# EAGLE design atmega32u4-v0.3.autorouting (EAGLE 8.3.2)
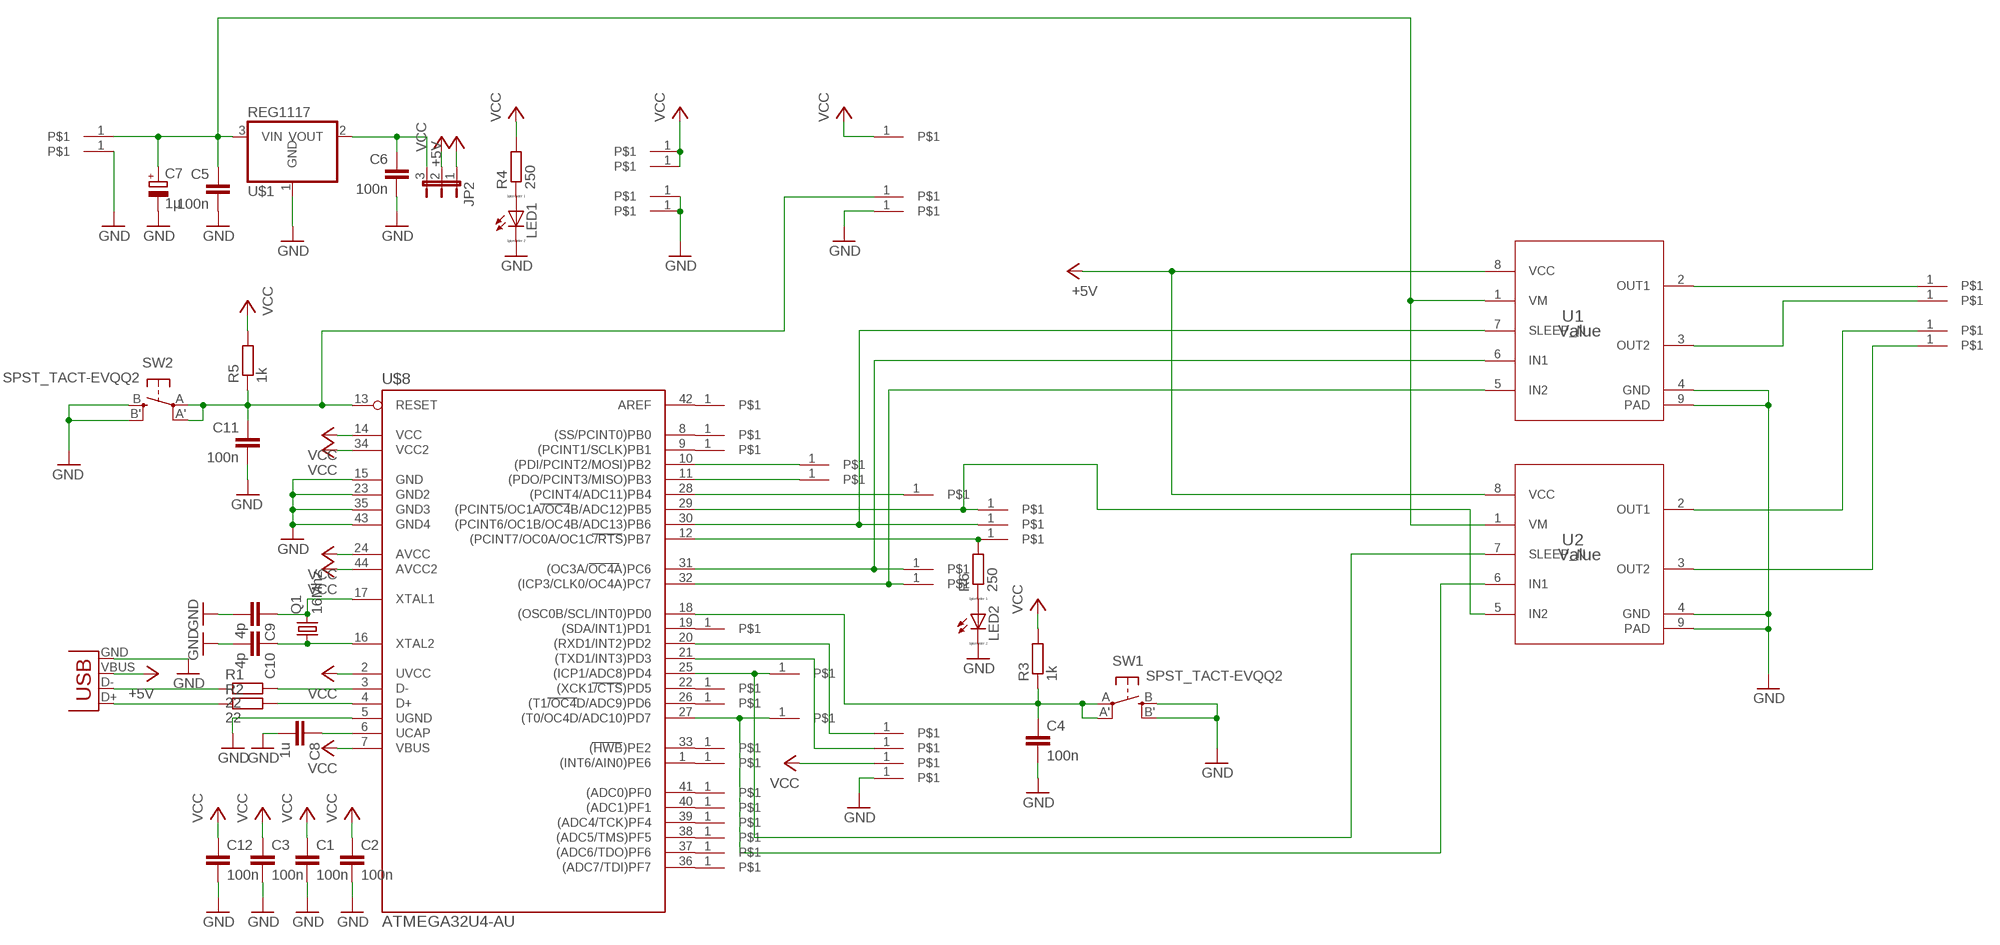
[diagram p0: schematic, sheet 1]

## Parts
C1  100n  C-EUC1206  [C1206]
C2  100n  C-EUC1206  [C1206]
C3  100n  C-EUC1206  [C1206]
C4  100n  C-EUC1206  [C1206]
C5  100n  C-EUC1206  [C1206]
C6  100n  C-EUC1206  [C1206]
C7  1µ  CPOL-EUC/6032-28R  [C/6032-28R]
C8  1u  C-EUC1206  [C1206]
C9  4p  C-EUC1206  [C1206]
C10  4p  C-EUC1206  [C1206]
C11  100n  C-EUC1206  [C1206]
C12  100n  C-EUC1206  [C1206]
JP2  JP2E  [JP2]
LED1  LED_E  [LED_1206]
LED2  LED_E  [LED_1206]
Q1  16Mhz  CRYSTALCTS406  [CTS406]
R1  22  R-EU_R1210  [R1210]
R2  22  R-EU_R1210  [R1210]
R3  1k  R-EU_R1210  [R1210]
R4  250  R-EU_R1210  [R1210]
R5  1k  R-EU_R1210  [R1210]
R6  250  R-EU_R1210  [R1210]
SW1  SPST_TACT-EVQQ2  [EVQ-Q2]
SW2  SPST_TACT-EVQQ2  [EVQ-Q2]
U1  Value  DRV8837DSGR  [DSG0008A]
U2  Value  DRV8837DSGR  [DSG0008A]
U$1  REG1117  [SOT223]
U$2  PIN1X1  [1X01]
U$3  PIN1X1  [1X01]
U$4  PIN1X1  [1X01]
U$5  PIN1X1  [1X01]
U$6  PIN1X1  [1X01]
U$7  PIN1X1  [1X01]
U$8  ATMEGA32U4-AU  [TQFP44]
U$9  PIN1X1  [1X01]
U$10  PIN1X1  [1X01]
U$11  PIN1X1  [1X01]
U$12  PIN1X1  [1X01]
U$13  PIN1X1  [1X01]
U$14  PIN1X1  [1X01]
U$15  PIN1X1  [1X01]
U$16  PIN1X1  [1X01]
U$17  PIN1X1  [1X01]
U$18  PIN1X1  [1X01]
U$19  PIN1X1  [1X01]
U$20  PIN1X1  [1X01]
U$21  PIN1X1  [1X01]
U$22  PIN1X1  [1X01]
U$23  PIN1X1  [1X01]
U$24  PIN1X1  [1X01]
U$25  PIN1X1  [1X01]
U$26  PIN1X1  [1X01]
U$27  PIN1X1  [1X01]
U$28  PIN1X1  [1X01]
U$29  PIN1X1  [1X01]
U$30  PIN1X1  [1X01]
U$31  PIN1X1  [1X01]
U$32  PIN1X1  [1X01]
U$38  PIN1X1  [1X01]
U$39  PIN1X1  [1X01]
U$40  PIN1X1  [1X01]
U$41  PIN1X1  [1X01]
U$42  PIN1X1  [1X01]
U$43  PIN1X1  [1X01]
U$44  PIN1X1  [1X01]
U$45  PIN1X1  [1X01]
U$46  PIN1X1  [1X01]
U$47  PIN1X1  [1X01]
U$48  PIN1X1  [1X01]
U$50  USB  [USB-MINIB]

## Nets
+5V: JP2.1 U$50.VBUS
GND: C1.2 C2.2 C3.2 C4.2 C5.2 C6.2 C7.- C8.2 C9.2 C10.2 C11.2 C12.2 LED1.C LED2.C SW1.B'(S1) SW1.B(S) SW2.B'(S1) SW2.B(S) U1.4(GND) U1.9(PAD) U2.4(GND) U2.9(PAD) U$1.1(GND) U$3.1 U$4.1 U$5.1 U$8.5(UGND) U$8.15(GND) U$8.23(GND2) U$8.35(GND3) U$8.43(GND4) U$11.1 U$32.1 U$50.GND
MISO: U$8.11((PDO/PCINT3/MISO)PB3) U$14.1
N$1: C5.1 C7.+ U1.1(VM) U2.1(VM) U$1.3(VIN) U$2.1
N$2: C6.1 JP2.3 U$1.2(VOUT)
N$3: LED1.A R4.1
N$4: U$8.19((SDA/INT1)PD1) U$21.1
N$5: U$8.42(AREF) U$48.1
N$6: LED2.A R6.1
N$7: U1.2(OUT1) U$31.1
N$8: U1.3(OUT2) U$30.1
N$9: U2.2(OUT1) U$29.1
N$10: U2.3(OUT2) U$22.1
N$11: U$8.28((PCINT4/ADC11)PB4) U$15.1
N$12: U2.6(IN1) U$8.27((T0/OC4D/ADC10)PD7) U$39.1
N$13: U2.5(IN2) U$8.29((PCINT5/OC1A/OC4B/ADC12)PB5) U$16.1
N$15: U1.7(SLEEP_N) U$8.30((PCINT6/OC1B/OC4B/ADC13)PB6) U$17.1
N$16: R6.2 U$8.12((PCINT7/OC0A/OC1C/RTS)PB7) U$18.1
N$17: U$8.8((SS/PCINT0)PB0) U$9.1
N$20: U1.5(IN2) U$8.32((ICP3/CLK0/OC4A)PC7) U$20.1
N$21: U1.6(IN1) U$8.31((OC3A/OC4A)PC6) U$19.1
N$23: U$8.10((PDI/PCINT2/MOSI)PB2) U$13.1
N$35: U2.7(SLEEP_N) U$8.25((ICP1/ADC8)PD4) U$26.1
N$36: U$8.22((XCK1/CTS)PD5) U$27.1
N$37: U$8.26((T1/OC4D/ADC9)PD6) U$38.1
N$44: U$8.33((HWB)PE2) U$40.1
N$45: U$8.1((INT6/AIN0)PE6) U$41.1
N$51: U$8.41((ADC0)PF0) U$42.1
N$52: U$8.40((ADC1)PF1) U$43.1
N$53: U$8.39((ADC4/TCK)PF4) U$44.1
N$54: U$8.38((ADC5/TMS)PF5) U$45.1
N$55: U$8.37((ADC6/TDO)PF6) U$46.1
N$56: U$8.36((ADC7/TDI)PF7) U$47.1
N$62: R2.1 U$50.D+
N$63: R1.1 U$50.D-
N$64: R1.2 U$8.3(D-)
N$65: R2.2 U$8.4(D+)
N$66: C8.1 U$8.6(UCAP)
N$67: C9.1 Q1.3 U$8.17(XTAL1)
N$68: C10.1 Q1.1 U$8.16(XTAL2)
RST: C11.1 R5.1 SW2.A'(P1) SW2.A(P) U$8.13(RESET) U$28.1
RST1: C4.1 R3.1 SW1.A'(P1) SW1.A(P) U$8.18((OSC0B/SCL/INT0)PD0)
RXD: U$8.20((RXD1/INT2)PD2) U$24.1
SCK: U$8.9((PCINT1/SCLK)PB1) U$12.1
TXD: U$8.21((TXD1/INT3)PD3) U$25.1
VCC: C1.1 C2.1 C3.1 C12.1 JP2.2 R3.2 R4.2 R5.2 U1.8(VCC) U2.8(VCC) U$6.1 U$7.1 U$8.2(UVCC) U$8.7(VBUS) U$8.14(VCC) U$8.24(AVCC) U$8.34(VCC2) U$8.44(AVCC2) U$10.1 U$23.1 ; supply symbol labelled +5V

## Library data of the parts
C1-C6 C8-C12 = rcl:C-EU: CAPACITOR, European symbol
C7 = rcl:CPOL-EU: POLARIZED CAPACITOR, European symbol
JP2 = jumper:JP2E: JUMPER
LED1 LED2 = eagle-ltspice:LED_E: LED; SPICEMODEL: NONE; SPICEPREFIX: D; SPICETYPE: diode
Q1 = beagle:CRYSTAL
R1-R6 = rcl:R-EU_: RESISTOR, European symbol
SW1 SW2 = adafruit:SPST_TACT: SMT 6mm switch, EVQQ2 series http://www.ladyada.net/library/eagle
U1 U2 = DRV8837:DRV8837DSGR; MANUFACTURER: Texas Instruments; PARTNUMBER: DRV8837DSGR; REFDES: RefDes; TYPE: TYPE
U$1 = CEDT:REG1117: 800mA and 1A Low Dropout (LDO) Positive Regulator 1.8V, 2.5V, 2.85V, 3.3V, 5V, and Adj
U$2-U$7 U$9-U$32 U$38-U$48 = beagle:PIN1X1
U$8 = mega32U4:ATMEGA32U4-AU
U$50 = beagle:USB

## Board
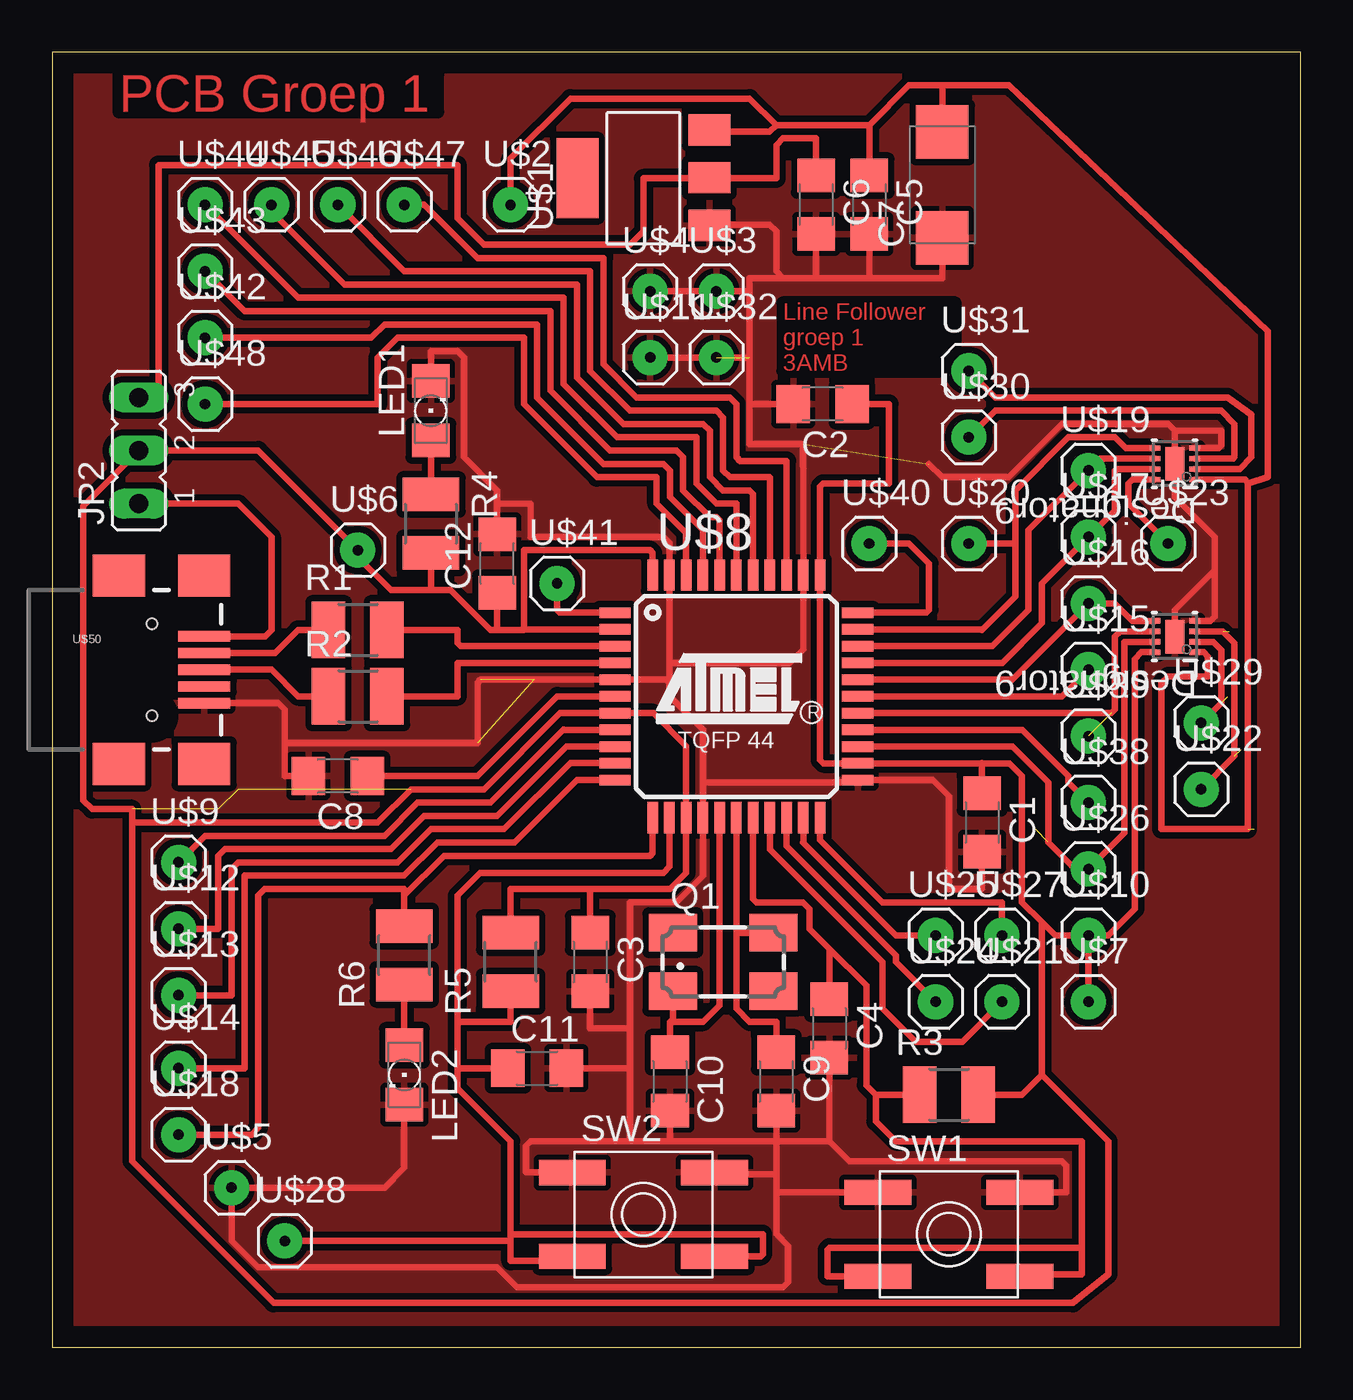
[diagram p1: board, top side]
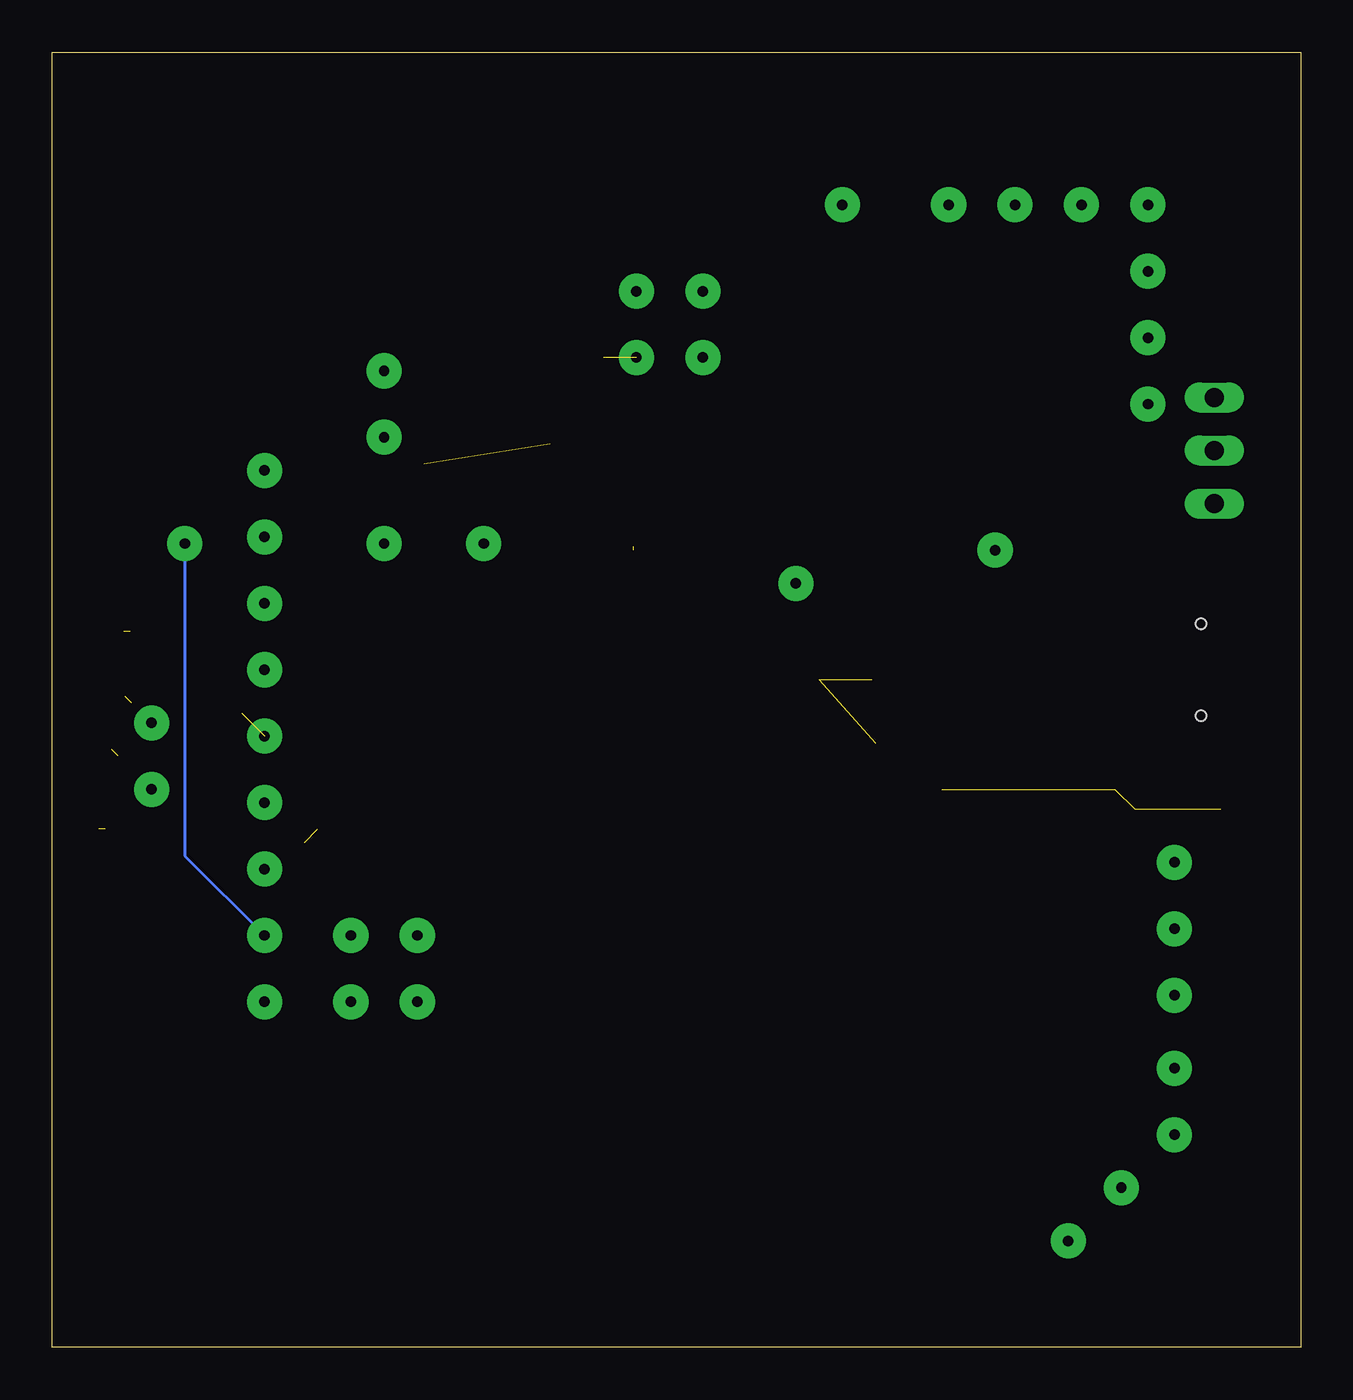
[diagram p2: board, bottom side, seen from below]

Size 59.68 x 61.9 mm. Coordinates in mm from the lower left corner, seen from the top.
Outline: 0,0 59.68,0 59.68,61.9 0,61.9 0,0
Copper layers (1*16): Top 0.035mm / dielectric 1.5mm / Bottom 0.035mm
Design rules "default": minimum track width 6mil, minimum drill 0.35mm, track to track 6mil, track to pad 6mil, pad to pad 6mil, via to via 6mil, smd to smd 6mil, copper to edge 40mil, drill to drill 6mil, minimum pad ring 10mil, minimum via ring 8mil, stop-mask expansion 4mil, vias tented up to drill 0mil, thermal gap 10mil

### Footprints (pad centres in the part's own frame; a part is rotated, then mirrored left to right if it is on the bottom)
C1206 = smd 1.6 x 1.8: 1 -1.4,0; 2 1.4,0
C/6032-28R = smd 2.55 x 2.5: + 2.525,0; - -2.525,0
JP2 = drill 0.914 long: 1 -2.54,0; 2 0,0; 3 2.54,0
LED_1206 = smd 1.6 x 1.803: A -1.422,0; C 1.422,0
CTS406 = smd 2.3 x 1.8: 1 -2.4,-1.4; 2 2.4,-1.4; 3 2.4,1.4; 4 -2.4,1.4
R1210 = smd 1.6 x 2.7: 1 -1.4,0; 2 1.4,0
EVQ-Q2 = smd 3.2 x 1.2: A -3.4,-2; A' 3.4,-2; B -3.4,2; B' 3.4,2
DSG0008A = smd 0.5 x 0.25: 1 -0.95,0.75; 2 -0.95,0.25; 3 -0.95,-0.25; 4 -0.95,-0.75; 5 0.95,-0.75; 6 0.95,-0.25; 7 0.95,0.25; 8 0.95,0.75 | smd 0.9 x 1.6: 9 0,0 | smd 0.5 x 0.5: V 0,-0.4
SOT223 = smd 1.499 x 2.007: 1 -2.261,-3.15; 2 0.025,-3.15; 3 2.311,-3.15 | smd 3.81 x 2.007: 4 0,3.15
1X01 = drill 0.5 pad 1.676: 1 0,0
TQFP44 = smd 1.5 x 0.5: 1 -5.8,4; 2 -5.8,3.2; 3 -5.8,2.4; 4 -5.8,1.6; 5 -5.8,0.8; 6 -5.8,0; 7 -5.8,-0.8; 8 -5.8,-1.6; 9 -5.8,-2.4; 10 -5.8,-3.2; 11 -5.8,-4; 23 5.8,-4; 24 5.8,-3.2; 25 5.8,-2.4; 26 5.8,-1.6; 27 5.8,-0.8; 28 5.8,0; 29 5.8,0.8; 30 5.8,1.6; 31 5.8,2.4; 32 5.8,3.2; 33 5.8,4 | smd 0.5 x 1.5: 12 -4,-5.8; 13 -3.2,-5.8; 14 -2.4,-5.8; 15 -1.6,-5.8; 16 -0.8,-5.8; 17 0,-5.8; 18 0.8,-5.8; 19 1.6,-5.8; 20 2.4,-5.8; 21 3.2,-5.8; 22 4,-5.8; 34 4,5.8; 35 3.2,5.8; 36 2.4,5.8; 37 1.6,5.8; 38 0.8,5.8; 39 0,5.8; 40 -0.8,5.8; 41 -1.6,5.8; 42 -2.4,5.8; 43 -3.2,5.8; 44 -4,5.8
USB-MINIB = smd 2.5 x 0.5: D+ 7.58,0; D- 7.58,0.8; GND 7.58,-1.6; ID 7.58,-0.8; VBUS 7.58,1.6 | smd 2.5 x 2: GND@1 3.5,-4.5; GND@2 3.5,4.5; GND@3 7.58,4.5; GND@4 7.58,-4.5 | hole 0.5: 5.08,2.2; 5.08,-2.2

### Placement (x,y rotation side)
C1  44.45,25.08 270 top
C2  36.83,45.09 180 top
C3  25.72,18.42 270 top
C4  37.15,15.24 270 top
C5  39.05,54.61 270 top
C6  36.51,54.61 270 top
C7  42.55,55.56 90 top
C8  13.65,27.31 180 top
C9  34.61,12.7 270 top
C10  29.53,12.7 270 top
C11  23.18,13.33 0 top
C12  21.27,37.46 90 top
JP2  4.13,42.86 90 top
LED1  18.1,44.77 90 top
LED2  16.83,13.02 270 top
Q1  32.07,18.42 0 top
R1  14.61,34.29 0 top
R2  14.61,31.12 0 top
R3  42.86,12.06 0 top
R4  18.1,39.37 270 top
R5  21.91,18.42 90 top
R6  16.83,18.73 90 top
SW1  42.86,5.4 0 top
SW2  28.26,6.35 0 top
U1  53.66,42.23 180 top
U2  53.66,33.97 180 top
U$1  28.26,55.88 90 top
U$2  21.91,54.61 0 top
U$3  31.75,50.48 0 top
U$4  28.57,50.48 0 top
U$5  8.57,7.62 0 top
U$6  14.61,38.1 0 top
U$7  49.53,16.51 0 top
U$8  32.7,31.12 0 top
U$9  6.03,23.18 0 top
U$10  49.53,19.69 0 top
U$11  28.57,47.31 0 top
U$12  6.03,20 0 top
U$13  6.03,16.83 0 top
U$14  6.03,13.33 0 top
U$15  49.53,32.38 0 top
U$16  49.53,35.56 0 top
U$17  49.53,38.73 0 top
U$18  6.03,10.16 0 top
U$19  49.53,41.91 0 top
U$20  43.82,38.42 0 top
U$21  45.4,16.51 0 top
U$22  54.93,26.67 0 top
U$23  53.34,38.42 0 top
U$24  42.23,16.51 0 top
U$25  42.23,19.69 0 top
U$26  49.53,22.86 0 top
U$27  45.4,19.69 0 top
U$28  11.11,5.08 0 top
U$29  54.93,29.85 0 top
U$30  43.82,43.5 0 top
U$31  43.82,46.67 0 top
U$32  31.75,47.31 0 top
U$38  49.53,26.04 0 top
U$39  49.53,29.21 0 top
U$40  39.05,38.42 0 top
U$41  24.13,36.51 0 top
U$42  7.3,48.26 0 top
U$43  7.3,51.43 0 top
U$44  7.3,54.61 0 top
U$45  10.48,54.61 0 top
U$46  13.65,54.61 0 top
U$47  16.83,54.61 0 top
U$48  7.3,45.09 0 top
U$50  -0.32,32.38 0 top

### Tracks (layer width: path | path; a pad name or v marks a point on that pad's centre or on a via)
+5V
  Top 0.305: U$50.VBUS 10.17,33.98 10.48,34.29 10.48,38.73 8.89,40.32 JP2.1
GND  (4 unrouted)
  Top 0.305: 37.15,9.84 C4.2 | U$50.GND 10.81,30.79 11.11,30.48 11.11,28.89 | 11.11,28.89 11.11,27.31 C8.2 | 27.62,15.24 27.62,13.33 | 27.62,15.24 27.62,21.27 29.84,21.27 31.1,22.53 U$8.15 31.1,26.99 | 27.62,13.33 27.62,9.84 | 29.53,9.84 27.62,9.84 | 34.61,9.84 29.53,9.84 | 34.61,9.84 C9.2 | C10.2 29.53,9.84 | C11.2 27.62,13.33 | C3.2 25.72,15.24 27.62,15.24 | 34.61,9.84 37.15,9.84 | 34.61,8.26 34.61,9.84 | 27.62,9.84 22.86,9.84 22.64,9.62 22.64,8.35 SW2.B | C1.2 44.45,21.91 42.86,21.91 42.86,26.35 42.1,27.12 U$8.23 38.37,26.99 31.1,26.99 | SW1.B' 48.48,7.4 48.48,8.67 48.26,8.89 38.1,8.89 37.15,9.84 | 21.27,40.32 C12.2 | 21.27,40.32 22.86,40.32 22.86,38.73 29.21,38.73 29.5,38.44 U$8.43 29.5,32.7 | 33.34,45.09 33.34,43.18 35.88,43.18 35.9,40.93 U$8.35 35.9,33.36 35.24,32.7 29.5,32.7 | 33.34,45.09 C2.2 | LED1.C 18.1,47.62 19.37,47.62 19.68,47.31 19.68,42.54 21.27,40.96 21.27,40.32 | 36.51,51.12 C6.2 | 39.05,51.12 36.51,51.12 | 39.05,51.12 C5.2 | C7.- 42.54,51.12 39.05,51.12 | U$1.1 31.45,53.66 34.29,53.66 34.61,53.34 34.61,51.43 34.93,51.12 | 34.93,51.12 36.51,51.12 | LED2.C 16.83,8.57 15.87,7.62 U$5.1 8.57,5.08 9.84,3.81 21.27,3.81 22.22,2.86 34.93,2.86 35.16,3.09 35.16,4.86 34.61,5.41 34.61,7.3 | 33.34,50.48 33.34,47.31 | 33.34,47.31 33.34,45.09 | 33.34,50.48 33.34,51.12 34.93,51.12 | 33.34,50.48 U$3.1 U$4.1 | 33.34,47.31 U$11.1 | 11.11,28.89 20.32,28.89 20.32,31.75 20.49,31.92 U$8.5 29.34,31.92 29.5,31.75 | 31.1,26.99 31.1,29.54 29.5,31.14 29.5,31.75 | 29.5,31.75 29.5,32.7 | U1.4 55.76,42.98 55.88,43.09 55.88,43.81 53.66,43.81 | 53.66,43.81 U1.9 53.66,40.64 55.56,38.73 55.56,37.15 | 55.56,37.15 53.66,35.24 U2.9
  Top 0.305: U2.4 55.36,34.72 55.56,34.92 55.56,37.15 | 53.66,43.81 53.34,44.13 48.26,44.13 45.72,41.59 42.54,41.59 41.91,42.23 | 34.61,7.3 34.61,8.26 | SW2.B' 31.75,8.26 34.61,8.26 | 34.61,7.3 34.7,7.4 SW1.B
  pour Top (isolate 0.305): -1.27,62.86 -1.27,-0.95 20.32,-0.95 60.33,-0.95 60.33,62.86
MISO
  Top 0.305: U$8.11 25.08,27.12 22.1,24.13 18.42,24.13 16.83,22.54 9.21,22.54 9.21,13.33 U$14.1
N$1  (1 unrouted)
  Top 0.305: U$1.3 31.5,58.1 34.29,58.1 34.61,58.42 | 39.05,58.42 34.61,58.42 | 39.05,58.42 C5.1 | C7.+ 42.54,60.32 | 42.54,60.32 40.96,60.32 39.05,58.42 | U$2.1 21.91,56.83 24.77,59.69 33.34,59.69 34.61,58.42 | 42.54,60.32 45.72,60.32 58.1,48.58 58.1,41.59 57.15,41.27 | U1.1 57.04,41.48 57.15,41.27 | U2.1 55.04,33.22 55.25,33.02 55.25,32.07 53.34,32.07 53.02,31.75 53.02,24.77 57.15,24.77 57.15,41.27
N$2
  Top 0.305: C6.1 36.51,57.78 34.93,57.78 34.61,57.47 34.61,55.88 31.43,55.88 U$1.2 31.38,55.88 28.26,55.88 28.26,53.34 27.62,52.7 20.64,52.7 19.37,53.98 19.37,56.52 5.08,56.52 5.08,45.4 JP2.3
N$3
  Top 0.305: LED1.A R4.1
N$4
  Top 0.305: U$8.19 34.3,23.8 39.69,18.42 39.69,16.19 41.28,14.61 43.5,14.61 U$21.1
N$5
  Top 0.305: U$48.1 15.56,45.09 15.56,47.31 16.51,48.26 22.54,48.26 22.54,45.09 26.04,41.59 28.89,41.59 28.89,40.32 30.3,38.91 U$8.42
N$6
  Top 0.305: R6.1 LED2.A
N$7
  Top 0.305: U1.2 56.76,41.98 57.33,42.54 57.33,44.59 56.2,45.4 45.08,45.4 U$31.1
N$8
  Top 0.305: U1.3 56.45,42.48 56.51,42.54 56.51,44.13 55.88,44.77 45.08,44.77 U$30.1
N$9  (1 unrouted)
  Top 0.305: U$29.1 55.88,30.8 55.88,33.34 55.5,33.72 U2.2
N$10  (2 unrouted)
  Top 0.305: U2.3 55.95,34.22 56.51,33.66 56.51,28.26 U$22.1
N$11
  Top 0.305: U$15.1 48.26,31.12 U$8.28
N$12  (1 unrouted)
  Top 0.305: U2.6 51.05,34.22 50.8,33.97 50.8,30.48 50.64,30.32 U$8.27
N$13
  Top 0.305: U$8.29 45.89,31.92 U$16.1 50.8,35.56 51.64,34.72 U2.5
N$15
  Top 0.305: U$8.30 45.41,32.71 47.31,34.61 47.31,36.51 U$17.1 50.8,40 50.8,41.91 50.87,41.98 U1.7
N$16
  Top 0.305: 16.83,21.59 16.83,21.91 10.16,21.91 9.84,21.59 9.84,10.48 9.52,10.16 U$18.1 | 16.83,21.59 R6.2 | U$8.12 28.7,23.62 28.58,23.5 18.73,23.5 16.83,21.59
N$17
  Top 0.305: U$9.1 7.3,24.45 15.87,24.45 17.46,26.04 20.95,26.04 24.45,29.53 24.46,29.52 U$8.8
N$20
  Top 0.305: U$8.32 44.43,34.31 44.45,34.29 46.04,35.88 46.04,38.42 | 46.04,38.42 46.04,40.96 48.58,43.5 50.8,43.5 51.32,42.98 U1.5 | U$20.1 46.04,38.42
N$21
  Top 0.305: U$8.31 40.96,33.52 41.14,33.52 44.94,33.52 46.67,35.24 46.67,39.05 U$19.1 50.1,42.48 U1.6
N$23
  Top 0.305: U$13.1 8.57,16.83 8.57,22.86 8.89,23.18 16.51,23.18 18.1,24.77 21.59,24.77 24.77,27.94 26.88,27.94 U$8.10
N$35  (1 unrouted)
  Top 0.305: U2.7 51.26,33.72 51.26,24.59 U$26.1 48.9,22.86 47.62,24.13 47.62,26.99 45.9,28.71 U$8.25
N$36
  Top 0.305: U$27.1 45.4,21.27 39.69,21.27 36.7,24.26 U$8.22 36.7,25.21
N$37
  Top 0.305: U$38.1 48.58,26.99 48.58,27.31 46.37,29.52 U$8.26
N$44
  Top 0.305: U$8.33 41.78,35.11 41.91,35.24 41.91,37.46 40.96,38.42 U$40.1
N$45
  Top 0.305: U$8.1 24.26,35.11 24.13,35.24 U$41.1
N$51
  Top 0.305: U$8.41 31.1,39.06 29.53,40.64 29.53,41.91 29.21,42.23 26.35,42.23 23.18,45.4 23.18,48.89 15.87,48.89 15.24,48.26 U$42.1
N$52  (1 unrouted)
  Top 0.305: U$8.40 31.9,38.27 | 7.62,51.43 U$43.1 9.21,49.53 23.81,49.53 23.81,45.72 26.67,42.86 29.84,42.86 30.16,42.54 30.16,40.96 31.43,39.69 31.75,39.69 31.9,39.53 31.9,38.1
N$53
  Top 0.305: 7.43,54.61 U$44.1 11.75,50.16 24.45,50.16 24.45,46.04 26.99,43.5 30.8,43.5 30.8,41.27 31.75,40.32 32.7,40.32 U$8.39
N$54
  Top 0.305: U$8.38 33.5,40.79 33.34,40.96 32.07,40.96 31.43,41.59 31.43,43.81 31.11,44.13 27.31,44.13 25.08,46.35 25.08,50.8 13.97,50.8 10.48,54.29 U$45.1
N$55
  Top 0.305: U$46.1 16.83,51.43 25.72,51.43 25.72,46.67 27.62,44.77 31.75,44.77 32.07,44.45 32.07,41.91 32.39,41.59 34.29,41.59 34.3,41.58 U$8.37
N$56
  Top 0.305: U$8.36 35.1,42.37 32.88,42.37 32.7,42.54 32.7,45.09 32.39,45.4 27.94,45.4 26.35,46.99 26.35,52.07 20.32,52.07 17.78,54.61 U$47.1 16.91,54.61
N$62
  Top 0.305: U$50.D+ 10.48,32.38 11.75,31.12 R2.1
N$63
  Top 0.305: U$50.D- 10.64,33.18 11.75,34.29 R1.1
N$64
  Top 0.305: R1.2 19.37,34.29 19.37,33.66 19.51,33.52 U$8.3
N$65
  Top 0.305: U$8.4 20.02,32.71 20,32.7 19.37,32.7 19.37,31.12 R2.2
N$66
  Top 0.305: U$8.6 24.13,31.12 20.32,27.31 C8.1
N$67
  Top 0.305: C9.1 34.61,15.56 33.34,15.56 32.7,16.19 32.7,19.69 | 32.7,19.69 32.7,24.45 | 32.7,24.45 32.7,24.77 | Q1.3 32.83,19.82 32.7,19.69 | 32.7,24.45 U$8.17
N$68
  Top 0.305: U$8.16 31.9,16.35 31.11,15.56 29.53,15.56 | 29.53,15.56 C10.1 | Q1.1 29.67,15.7 29.53,15.56
RST
  Top 0.305: R5.1 21.91,15.56 19.37,15.56 | 19.37,13.33 19.37,15.56 | 19.37,13.33 C11.1 | 19.37,15.56 19.37,21.59 20.16,22.38 | 20.16,22.38 20.46,22.68 | U$8.13 29.5,22.98 29.21,22.68 20.46,22.68 | 21.91,5.08 21.91,4.13 24.63,4.13 SW2.A | 21.91,5.4 21.91,5.08 | 21.91,5.4 21.91,9.84 19.37,12.38 19.37,13.33 | U$28.1 21.91,5.08 | SW2.A' 33.88,4.35 33.97,4.45 33.97,5.4 21.91,5.4 | 20.46,22.68 20.16,22.38
RST1
  Top 0.305: U$8.18 33.5,21.43 33.65,21.27 35.88,21.27 36.19,20.96 36.19,20 37.15,19.05 | C4.1 37.15,19.05 | 37.15,19.05 38.91,17.29 38.91,12.52 39.37,12.06 | 39.37,12.06 R3.1 | 39.37,12.06 39.37,10.79 40.32,9.84 49.21,9.84 49.21,4.76 | 49.21,4.76 49.21,3.49 46.36,3.49 SW1.A' | SW1.A 37.05,3.4 37.05,4.67 37.15,4.76 49.21,4.76
RXD
  Top 0.305: U$8.20 35.1,23.95 40.32,18.73 40.32,18.42 U$24.1
SCK
  Top 0.305: U$12.1 7.94,20 7.94,23.5 8.26,23.81 16.19,23.81 17.78,25.4 21.27,25.4 24.59,28.71 U$8.9
TXD
  Top 0.305: U$8.21 35.9,24.16 35.88,24.13 40.32,19.69 U$25.1
VCC  (3 unrouted)
  Top 0.305: R5.2 21.91,21.91 25.72,21.91 | 44.43,27.92 U$8.24 36.86,27.92 36.7,28.07 U$8.34 36.7,41.15 36.83,41.27 40.01,41.27 40.01,45.09 C2.1 | 44.43,27.92 44.45,27.94 C1.1 | 44.43,27.92 45.75,27.92 46.36,27.31 46.36,21.27 47.31,20.32 | 47.31,13.02 46.36,12.06 R3.2 | 47.31,20.32 47.31,13.02 | U$8.2 22.54,34.31 | 22.54,34.31 22.54,38.1 28.58,38.1 28.7,37.97 U$8.44 | 21.27,34.29 20.95,34.29 19.05,36.2 18.1,36.2 | 18.1,36.2 R4.2 | 18.1,36.2 16.19,36.2 14.6,37.78 U$6.1 9.84,42.86 JP2.2 1.49,40.22 1.49,26.14 1.9,25.72 3.81,25.72 3.81,25.08 | C12.1 21.27,34.29 | 22.54,34.31 22.52,34.29 21.27,34.29 | 47.31,20.32 47.94,19.69 U$10.1 | U$10.1 U$7.1 | U$10.1 50.48,19.69 51.75,20.96 51.75,32.91 52.07,33.22 U2.8 | U1.8 51.64,41.48 51.43,41.27 51.43,40.32 U$23.1 | 47.31,13.02 50.48,9.84 50.48,3.49 48.79,2.12 10.58,2.12 3.81,8.89 3.81,25.08 | 25.72,21.91 29.53,21.91 30.3,22.68 U$8.14 30.3,28.75 28.74,30.32 U$8.7 24.28,30.32 20.64,26.67 17.15,26.67 15.56,25.08 3.81,25.08 | C3.1 25.72,21.91
  Bottom 0.152: U$23.1 53.34,23.5 U$10.1

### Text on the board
Top: PCB Groep 1 | Line Follower / groep 1 / 3AMB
